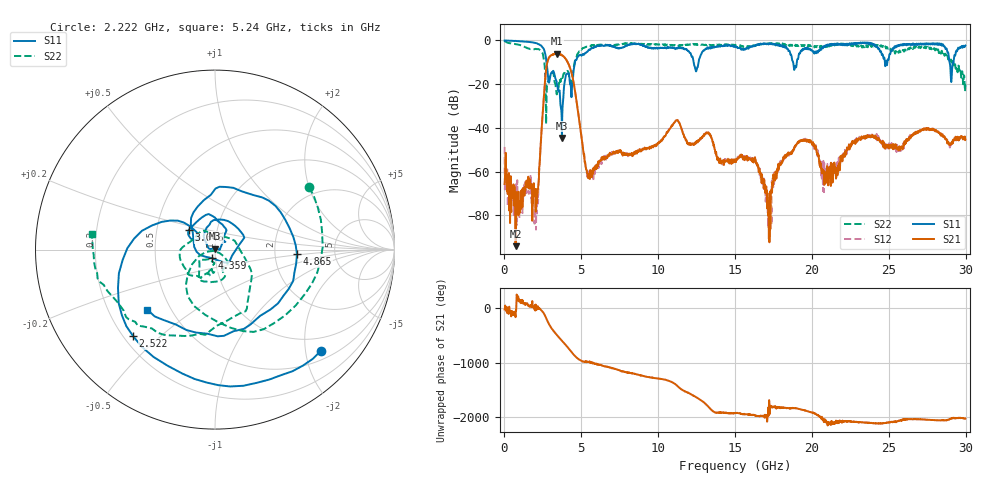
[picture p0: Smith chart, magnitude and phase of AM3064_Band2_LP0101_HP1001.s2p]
# Hz S DB R 50.0
!freq dBS11 angS11 dBS21 angS21 dBS12 angS12 dBS22 angS22
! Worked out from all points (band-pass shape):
!   1600 points, 10 MHz to 29.98 GHz, reference 50 ohm
!   highest |S21| = -6.00 dB at 3.403 GHz (marker M1); lowest = -94.1 dB at 722.3 MHz (marker M2)
!   |S21| within 3 dB of the highest: 2.832 GHz to 4.026 GHz (1.194 GHz wide, 34.8 % of centre)
!   lowest |S11| = -44.7 dB at 3.74 GHz (marker M3), VSWR 1.01, Z = 50 + j0.584 ohm
!   |S11| at or under -10 dB: 2.737 GHz to 4.589 GHz (1.852 GHz wide, 50.6 % of centre); 12.3 GHz to 12.62 GHz (325.2 MHz wide, 2.61 % of centre); 28.95 GHz to 29.2 GHz (253.8 MHz wide, 0.873 % of centre)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
!   |S22| runs from -38.2 to -0.2 dB; largest |S21 - S12| = 0.014
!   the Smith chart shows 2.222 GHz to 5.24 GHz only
!   S11 on the Smith chart (normalised r, x): 2.222 GHz: 0.69, -2.32; 2.522 GHz: 0.24, -0.41; 3.046 GHz: 0.73, +0.16; 4.359 GHz: 0.97, -0.09; 4.865 GHz: 2.67, -0.17; 5.24 GHz: 0.37, -0.33
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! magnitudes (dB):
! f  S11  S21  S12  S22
! 10 MHz  0.0  -65.8  -48.7  -0.2
! 722.3 MHz  -0.2  -94.1  -80.5  -1.7
! 2.222 GHz  -1.8  -65.0  -63.6  -4.0
! 2.522 GHz  -3.6  -29.8  -29.7  -7.0
! 3.046 GHz  -14.8  -6.7  -6.7  -15.0
! 3.403 GHz  -19.6  -6.0  -6.0  -24.7
! 3.74 GHz  -44.7  -6.8  -6.7  -16.7
! 4.359 GHz  -26.0  -14.8  -14.7  -20.8
! 4.865 GHz  -6.8  -36.4  -36.6  -5.0
! 5.015 GHz  -7.0  -44.4  -44.3  -4.2
! 5.24 GHz  -6.0  -55.5  -55.9  -3.2
! 10 GHz  -3.5  -47.3  -47.0  -1.9
! 11.22 GHz  -3.7  -36.5  -36.4  -2.3
! 15 GHz  -2.7  -55.6  -54.6  -2.0
! 16.34 GHz  -2.4  -54.9  -54.7  -2.4
! 17.22 GHz  -1.4  -80.5  -73.4  -1.5
! 18 GHz  -2.8  -56.0  -56.7  -1.7
! 19.99 GHz  -4.5  -47.0  -46.8  -2.2
! 20.95 GHz  -2.7  -59.9  -61.5  -2.4
! 23.1 GHz  -1.4  -45.0  -44.5  -2.5
! 25 GHz  -8.5  -48.0  -48.6  -3.3
! 29.98 GHz  -2.4  -45.3  -45.7  -20.2
